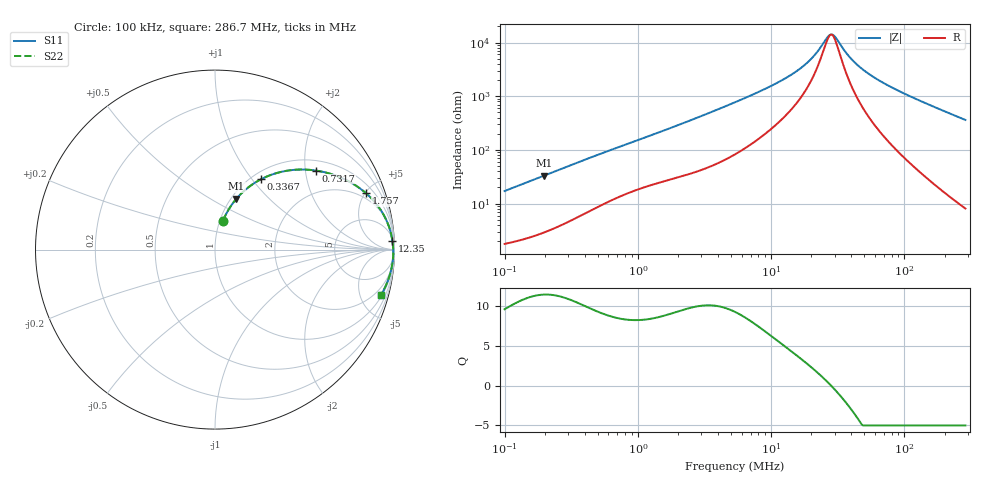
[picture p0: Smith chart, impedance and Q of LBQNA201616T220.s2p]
! LBQNA201616T220  S-PARAMETER MODEL  ( General Type )
! Model Generated by TAIYO YUDEN Corporation (http://www.ty-top.com)
! Version 1.0
! TAIYO YUDEN Control No. 191025NI43SB-FBB
! Copyright(c) 2019 TAIYO YUDEN CO.,LTD. All Rights Reserved.
! Product Description (link to TY-COMPAS)
! https://ds.yuden.co.jp/TYCOMPAS/or/detail?pn=LBQNA201616T220K&u=M
! Products Name : Inductors
! Characteristics :
!  Inductance : 22 uH , SRF(min) : 16 MHz , DC Resistance(max) : 1.3 Ohm
!  Rated Current : Saturation :165 mA , Temp Rise : 190 mA (20 degC)
!  Case Size : 2.0 x 1.6 / 0.079 x 0.063 [mm/inch] , Thickness : 1.6 / 0.063 [mm/inch]
!  (Conditions: Temperature = 25 degC , DC Bias Current/Voltage = 0A / 0V)
! External Node Assignments :
!  1  o---GGG---o  2
! GND o---------o GND
! Frequency Range : 0.1MHz  -  286.687601MHz  [ 402 STEP ]
# MHz S RI R 50
! Freq[MHz].  S11 Real  S11 Imag  S21 Real  S21 Imag  S12 Real  S12 Imag  S22 Real  S22 Imag
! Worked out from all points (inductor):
!   401 points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, 100 kHz to 286.7 MHz, reference 50 ohm
!   read as one part in series: L = 27 uH near 104.1 kHz
!   highest Q = 11.5 at 196.7 kHz (marker M1), where L = 26.8 uH
!   self-resonance near 27.93 MHz
!   S11 on the Smith chart (normalised r, x): 100 kHz: 1.04, +0.34; 336.7 kHz: 1.11, +1.11; 731.7 kHz: 1.27, +2.28; 1.757 MHz: 1.56, +5.09; 12.35 MHz: 9, +40; 286.7 MHz: 1.16, -7.23
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0.1  0.0444 0.1604  0.9556 -0.1604  0.9556 -0.1604  0.0444 0.1604
0.196734  0.1192 0.2833  0.8808 -0.2833  0.8808 -0.2833  0.1192 0.2833
0.336709  0.2572 0.3923  0.7428 -0.3923  0.7428 -0.3923  0.2572 0.3923
0.379416  0.299 0.4114  0.701 -0.4114  0.701 -0.4114  0.299 0.4114
0.532177  0.432 0.4436  0.568 -0.4436  0.568 -0.4436  0.432 0.4436
0.731732  0.5622 0.4404  0.4378 -0.4404  0.4378 -0.4404  0.5622 0.4404
1.439567  0.7928 0.3514  0.2072 -0.3514  0.2072 -0.3514  0.7928 0.3514
1.756577  0.8419 0.3136  0.1581 -0.3136  0.1581 -0.3136  0.8419 0.3136
2.889051  0.9252 0.2178  0.0748 -0.2178  0.0748 -0.2178  0.9252 0.2178
5.354322  0.9706 0.1234  0.0294 -0.1234  0.0294 -0.1234  0.9706 0.1234
12.35186  0.9885 0.0468  0.0115 -0.0468  0.0115 -0.0468  0.9885 0.0468
16.32081  0.9907 0.0295  0.00933 -0.0295  0.00933 -0.0295  0.9907 0.0295
20.31517  0.9919 0.0173  0.00814 -0.0173  0.00814 -0.0173  0.9919 0.0173
26.84292  0.9928 0.00257  0.00715 -0.00257  0.00715 -0.00257  0.9928 0.00257
29.06724  0.993 -0.00163  0.00697 0.00163  0.00697 0.00163  0.993 -0.00163
30.85563  0.9931 -0.00479  0.00686 0.00479  0.00686 0.00479  0.9931 -0.00479
37.6504  0.9933 -0.0156  0.00671 0.0156  0.00671 0.0156  0.9933 -0.0156
44.14869  0.9932 -0.0248  0.00685 0.0248  0.00685 0.0248  0.9932 -0.0248
56.05832  0.9924 -0.0399  0.00756 0.0399  0.00756 0.0399  0.9924 -0.0399
77.07906  0.9902 -0.0637  0.00983 0.0637  0.00983 0.0637  0.9902 -0.0637
140.0368  0.9779 -0.127  0.0221 0.127  0.0221 0.127  0.9779 -0.127
286.6876  0.9241 -0.2538  0.0759 0.2538  0.0759 0.2538  0.9241 -0.2538
